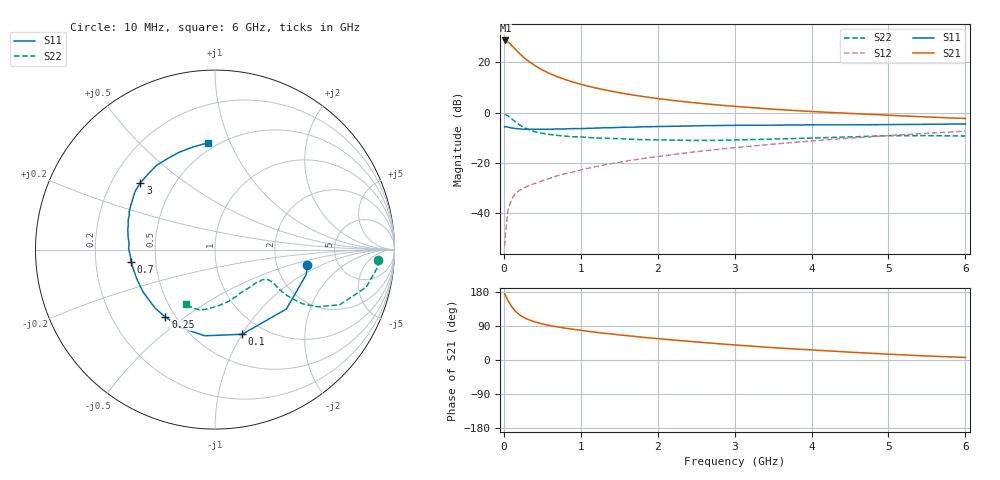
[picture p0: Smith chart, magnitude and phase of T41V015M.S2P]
! Infineon Technologies  Discrete & RF Semiconductors
! BFR182T
! Si NPN RF Bipolar Junction Transistor in SC75
! VCE = 1 V  IC = 15 mA
! Common Emitter S-Parameters:  October  1999
# GHz  S  MA  R  50
!  f  S11  S21  S12  S22
! GHz  MAG  ANG  MAG  ANG  MAG  ANG  MAG  ANG
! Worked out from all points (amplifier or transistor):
!   36 points, 10 MHz to 6 GHz, reference 50 ohm
!   highest |S21| = 28.7 dB at 20 MHz (marker M1)
!   |S21| within 3 dB of that: start of sweep to 133.8 MHz
!   unconditionally stable (mu >= 1): start of sweep to 11.42 MHz; 451.2 MHz to 5.192 GHz
!   at 250 MHz: K = 0.72, MSG = 26.2 dB, |S12| = -30.2 dB
!   at 1.4 GHz: K = 1.30, MAG = 11.1 dB, |S12| = -20.3 dB
!   at 6 GHz: K = 0.98, MSG = 2.5 dB, |S12| = -7.4 dB
!   S11 on the Smith chart (normalised r, x): 10 MHz: 2.98, -0.70; 100 MHz: 0.80, -1.00; 250 MHz: 0.44, -0.42; 700 MHz: 0.36, -0.07; 3 GHz: 0.32, +0.35; 6 GHz: 0.45, +0.83
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0.01  0.52 -9.5  27.28 174.6  0.0022 79.5  0.9096 -3.7
0.02  0.5275 -15.1  27.3 171.3  0.0036 82.9  0.9137 -5.8
0.05  0.5173 -39.8  25.75 158.4  0.0107 76.4  0.8682 -14.0
0.1  0.4955 -72.2  21.94 141.4  0.0191 64.7  0.7597 -23.9
0.15  0.4835 -96.7  18.18 128.6  0.0244 59.6  0.6527 -29.2
0.2  0.4754 -113.5  15.21 119.8  0.0281 57.4  0.5757 -31.7
0.25  0.4668 -126.3  12.9 113.3  0.0309 54.0  0.5145 -32.4
0.3  0.4667 -135.9  11.14 108.2  0.0341 55.2  0.474 -32.5
0.4  0.4652 -149.8  8.683 100.6  0.0389 56.4  0.4173 -31.7
0.5  0.4652 -159.1  7.082 95.3  0.044 58.6  0.3878 -30.3
0.6  0.4672 -166.0  5.95 90.9  0.0494 60.1  0.3671 -29.8
0.7  0.4726 -171.4  5.154 87.2  0.0556 62.2  0.3517 -29.4
0.9  0.4812 179.5  4.052 81.1  0.0658 64.6  0.331 -29.9
1.1  0.4876 172.3  3.348 75.5  0.0782 66.0  0.3199 -31.5
1.3  0.4995 166.6  2.863 70.7  0.0906 66.9  0.309 -33.7
1.6  0.5133 159.9  2.345 64.3  0.109 67.4  0.2973 -37.7
2.2  0.5348 149.9  1.747 52.8  0.1466 67.5  0.2846 -48.8
3  0.558 138.2  1.334 39.8  0.2011 65.1  0.2853 -64.8
3.5  0.5627 131.1  1.169 32.5  0.2358 62.7  0.2983 -75.3
4.5  0.5718 117.8  0.964 20.7  0.3105 56.4  0.3286 -94.8
5.5  0.5851 101.8  0.82 10.5  0.3883 48.9  0.3486 -110.9
6  0.5958 94.0  0.764 6.8  0.4274 44.3  0.3423 -118.2
